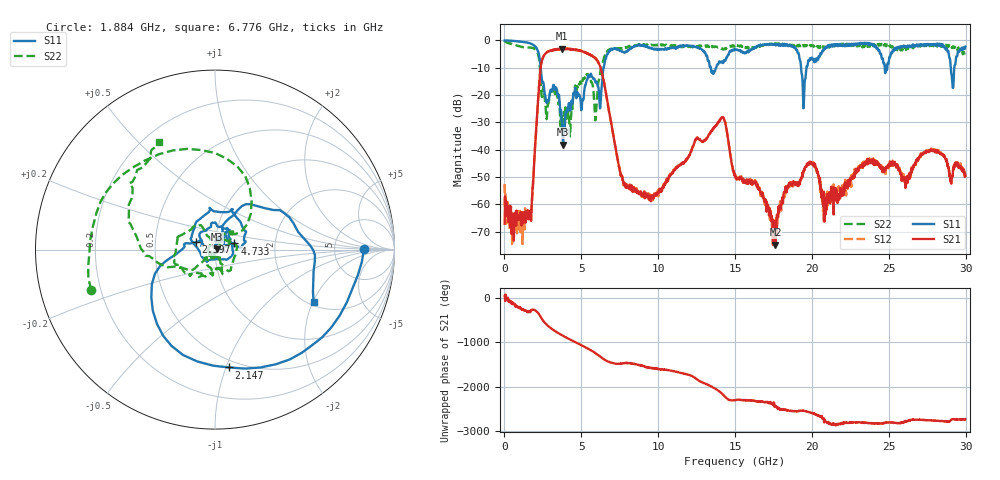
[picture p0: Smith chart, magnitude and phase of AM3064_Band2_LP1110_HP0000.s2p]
# Hz S DB R 50.0
!freq dBS11 angS11 dBS21 angS21 dBS12 angS12 dBS22 angS22
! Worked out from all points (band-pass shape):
!   1600 points, 10 MHz to 29.98 GHz, reference 50 ohm
!   highest |S21| = -3.03 dB at 3.759 GHz (marker M1); lowest = -74.7 dB at 17.63 GHz (marker M2)
!   |S21| within 3 dB of the highest: 2.526 GHz to 5.809 GHz (3.283 GHz wide, 78.8 % of centre)
!   lowest |S11| = -38.1 dB at 3.815 GHz (marker M3), VSWR 1.03, Z = 51.2 + j0.257 ohm
!   |S11| at or under -10 dB: 2.355 GHz to 6.452 GHz (4.097 GHz wide, 93 % of centre); 13.42 GHz to 13.77 GHz (344.9 MHz wide, 2.54 % of centre); 19.29 GHz to 19.64 GHz (348.7 MHz wide, 1.79 % of centre)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
!   |S22| runs from -35.1 to -0.2 dB; largest |S21 - S12| = 0.021
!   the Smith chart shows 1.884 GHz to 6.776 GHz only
!   S11 on the Smith chart (normalised r, x): 1.884 GHz: 11, +0; 2.147 GHz: 0.44, -1.03; 2.597 GHz: 0.80, +0.07; 4.733 GHz: 1.24, +0.09; 6.776 GHz: 2.14, -2.02
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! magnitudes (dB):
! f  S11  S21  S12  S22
! 10 MHz  0.0  -67.1  -52.6  -0.2
! 1.21 GHz  -0.6  -66.2  -66.9  -2.5
! 1.884 GHz  -1.6  -50.4  -49.3  -2.8
! 2.147 GHz  -3.6  -25.3  -25.1  -4.4
! 2.597 GHz  -18.9  -5.3  -5.3  -20.3
! 3.759 GHz  -32.0  -3.0  -3.1  -30.1
! 3.815 GHz  -38.1  -3.1  -3.0  -29.5
! 4.733 GHz  -18.9  -3.5  -3.5  -16.9
! 5.015 GHz  -25.1  -3.9  -3.9  -16.4
! 5.933 GHz  -15.4  -6.7  -6.7  -28.2
! 6.776 GHz  -4.1  -24.9  -24.9  -3.4
! 7.826 GHz  -4.4  -52.7  -52.9  -2.7
! 10 GHz  -3.4  -56.0  -57.1  -1.8
! 14.14 GHz  -7.8  -28.4  -28.3  -2.9
! 15 GHz  -3.1  -49.8  -49.7  -2.0
! 17.63 GHz  -1.8  -74.7  -69.0  -1.1
! 19.47 GHz  -24.1  -47.5  -47.9  -2.2
! 19.99 GHz  -6.3  -44.7  -44.8  -1.8
! 20.83 GHz  -3.2  -59.7  -62.0  -2.3
! 25 GHz  -7.9  -45.2  -45.0  -1.6
! 29.18 GHz  -17.4  -47.5  -47.6  -2.2
! 29.98 GHz  -2.3  -49.5  -49.4  -4.6
